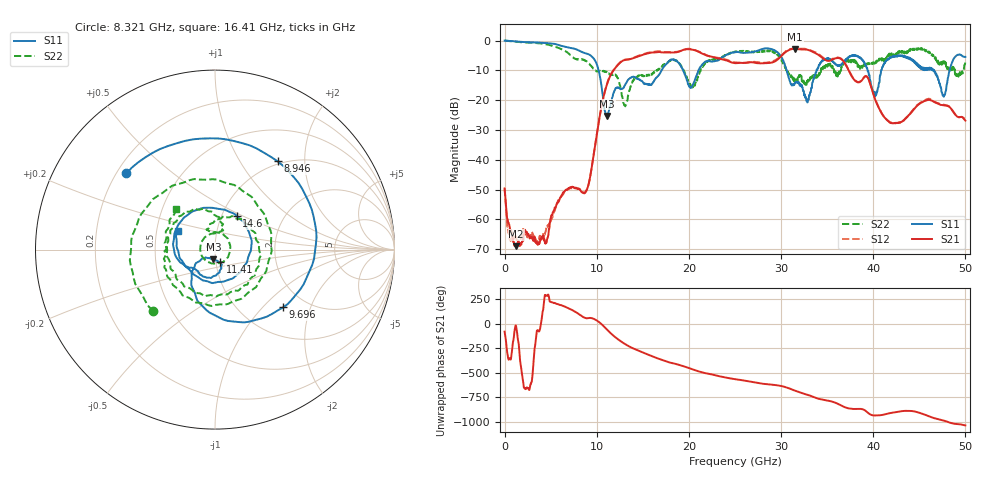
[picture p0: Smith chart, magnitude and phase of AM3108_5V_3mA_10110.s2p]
# Hz S DB R 50.0
!freq dBS11 angS11 dBS21 angS21 dBS12 angS12 dBS22 angS22
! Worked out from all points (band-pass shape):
!   1601 points, 10 MHz to 50 GHz, reference 50 ohm
!   highest |S21| = -2.76 dB at 31.53 GHz (marker M1); lowest = -69.0 dB at 1.26 GHz (marker M2)
!   |S21| within 3 dB of the highest: 14.06 GHz to 22.9 GHz (8.838 GHz wide, 47.8 % of centre); 29.83 GHz to 34.46 GHz (4.629 GHz wide, 14.4 % of centre)
!   lowest |S11| = -25.3 dB at 11.13 GHz (marker M3), VSWR 1.12, Z = 48.8 - j5.27 ohm
!   |S11| at or under -10 dB: 10.22 GHz to 17.03 GHz (6.815 GHz wide, 50 % of centre); 30.62 GHz to 33.85 GHz (3.227 GHz wide, 10 % of centre); 46.62 GHz to 48.29 GHz (1.667 GHz wide, 3.51 % of centre)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
!   |S22| runs from -22.1 to 0.1 dB; largest |S21 - S12| = 0.023
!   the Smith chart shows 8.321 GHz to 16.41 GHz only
!   S11 on the Smith chart (normalised r, x): 8.321 GHz: 0.24, +0.35; 8.946 GHz: 0.96, +1.48; 9.696 GHz: 1.54, -1.32; 11.41 GHz: 1.05, -0.15; 14.6 GHz: 1.18, +0.46; 16.41 GHz: 0.64, +0.14
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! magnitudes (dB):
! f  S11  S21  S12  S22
! 10 MHz  0.0  -49.6  -49.7  0.1
! 1.26 GHz  -0.3  -69.0  -66.3  -0.4
! 8.321 GHz  -3.7  -50.7  -50.3  -6.3
! 8.352 GHz  -3.7  -50.9  -50.5  -6.3
! 8.946 GHz  -4.4  -49.9  -50.0  -7.0
! 9.696 GHz  -6.1  -37.8  -37.8  -9.6
! 11.13 GHz  -25.3  -14.5  -14.3  -10.8
! 11.41 GHz  -22.4  -12.2  -12.1  -11.4
! 13.1 GHz  -14.7  -6.5  -6.4  -22.1
! 14.6 GHz  -13.0  -5.2  -5.0  -11.6
! 16.41 GHz  -12.7  -3.9  -3.7  -10.1
! 16.69 GHz  -11.7  -3.8  -3.6  -9.8
! 20.41 GHz  -14.8  -3.0  -3.0  -15.7
! 25 GHz  -3.9  -7.5  -7.3  -3.9
! 29.29 GHz  -3.2  -7.1  -6.7  -3.9
! 31.53 GHz  -14.2  -2.8  -2.7  -13.9
! 33.35 GHz  -15.6  -3.6  -3.4  -12.7
! 38 GHz  -4.9  -13.4  -13.3  -6.6
! 40.22 GHz  -18.7  -19.9  -19.7  -7.6
! 41.69 GHz  -6.0  -27.2  -27.1  -5.3
! 47.66 GHz  -18.8  -21.7  -21.6  -7.7
! 50 GHz  -5.4  -26.9  -26.4  -6.9
